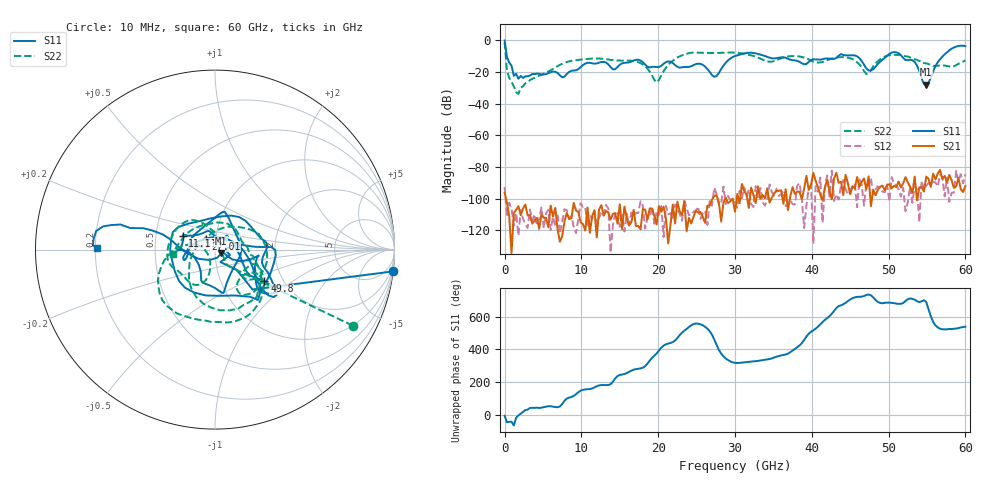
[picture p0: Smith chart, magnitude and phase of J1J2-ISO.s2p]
!Keysight Technologies,N5227A,US51270214,A.10.65.11
!Date: Thursday, October 15, 2020 07:30:32
!Correction: S11(Full 2 Port(1,2))
!S21(Full 2 Port(1,2))
!S12(Full 2 Port(1,2))
!S22(Full 2 Port(1,2))
!S2P File: Measurements: S11, S21, S12, S22:
# Hz S  dB  R 50
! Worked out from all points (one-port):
!   201 points, 10 MHz to 60 GHz, reference 50 ohm
!   lowest |S11| = -28.0 dB at 54.9 GHz (marker M1), VSWR 1.08, Z = 53.6 - j2.04 ohm
!   |S11| at or under -10 dB: 301.1 MHz to 29.94 GHz (29.64 GHz wide, 196 % of centre); 33.99 GHz to 43.44 GHz (9.442 GHz wide, 24.4 % of centre); 51.72 GHz to 57.06 GHz (5.342 GHz wide, 9.82 % of centre)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
!   S11 on the Smith chart (normalised r, x): 10 MHz: 0, -16; 11.11 GHz: 0.69, +0.11; 27.01 GHz: 0.89, +0.11; 49.8 GHz: 1.61, -0.64; 60 GHz: 0.21, +0.01
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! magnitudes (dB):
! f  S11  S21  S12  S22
! 10 MHz  0.0  -96.3  -92.6  -1.1
! 309.9 MHz  -10.3  -102.4  -111.5  -19.0
! 1.81 GHz  -24.2  -104.8  -123.2  -33.8
! 7.509 GHz  -23.3  -123.7  -114.2  -14.7
! 10.21 GHz  -15.6  -116.1  -105.3  -12.0
! 11.11 GHz  -14.2  -121.6  -110.6  -11.6
! 14.41 GHz  -18.2  -109.2  -109.7  -12.6
! 17.11 GHz  -12.3  -117.2  -109.1  -13.3
! 20.11 GHz  -16.8  -104.7  -110.2  -24.9
! 22.51 GHz  -16.6  -101.9  -105.5  -10.8
! 25.51 GHz  -14.8  -108.5  -112.8  -7.8
! 27.01 GHz  -21.8  -100.6  -104.5  -8.0
! 30 GHz  -9.9  -108.3  -102.1  -7.7
! 40.2 GHz  -11.9  -83.7  -128.4  -13.4
! 44.7 GHz  -9.5  -90.3  -97.3  -10.9
! 47.1 GHz  -17.7  -94.2  -90.1  -21.3
! 49.8 GHz  -9.7  -91.5  -90.9  -9.8
! 50.1 GHz  -8.5  -90.8  -101.9  -9.4
! 53.4 GHz  -13.6  -86.1  -92.1  -12.0
! 54.9 GHz  -28.0  -86.1  -91.7  -14.5
! 57.3 GHz  -8.8  -85.6  -98.6  -15.9
! 60 GHz  -3.6  -92.1  -84.6  -12.6
